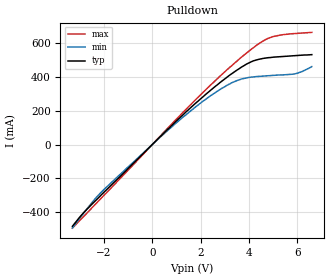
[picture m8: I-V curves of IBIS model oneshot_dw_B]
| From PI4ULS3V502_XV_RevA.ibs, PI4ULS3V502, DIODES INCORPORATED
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[Model]   oneshot_dw_B
Model_type  Open_sink
Vref = 3.3
Rref = 50
Vmeas = 1.65
C_comp   8.864pF   8.757pF   8.982pF
[Voltage Range]   3.30V   3.0V   3.6V
[Temperature Range]   25   85   -40
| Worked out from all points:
|   slope of the pulldown table from 0 to 0.495 V, typ, clamps not added: 7.05 ohm
[Pulldown]
-3.3V     -484mA     -494mA     -495mA
-2.5V     -354mA     -345mA     -376mA
-1.9V     -269mA     -253mA     -287mA
900mV     126mA      117mA      136mA
2.5V      332mA      298mA      364mA
3.1V      400mA      352mA      444mA
3.7V      460mA      389mA      519mA
4.2V      497mA      401mA      576mA
4.7V      513mA      407mA      623mA
5.3V      521mA      413mA      649mA
5.9V      527mA      419mA      658mA
6.6V      533mA      462mA      665mA
[Ramp]
| variable   typ   min   max
dV/dt_r   1.73/513.2E-12   1.56/511.7E-12   1.91/507.6E-12
dV/dt_f   1.73/112.1E-12   1.56/130.7E-12   1.91/97.4E-12
R_load = 50
